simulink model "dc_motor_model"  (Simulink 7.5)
settings: Solver=ode45  StartTime=0.0  StopTime=40  RelTol=1e-3
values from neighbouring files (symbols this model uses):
  K = 12/4000    (= 0.003)    [INITIAL_PARAM.m]
  k2 = 12/4000    (= 0.003)    [INITIAL_PARAM.m]
  R = 10    [INITIAL_PARAM.m]
libraries: fl_lib x10, nesl_utility x4

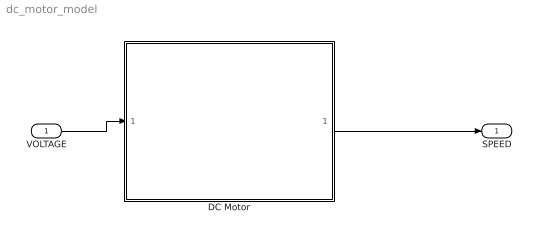
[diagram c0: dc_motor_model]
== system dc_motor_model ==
  VOLTAGE : Inport  OutDataType=fixdt(1, 16)  OutScaling=2^0
  DC Motor : Subsystem  mask{IMG='dcimaag.bmp'}
      mask prompts: IMG "Image File"
      mask init:
      | block=gcb;
      | img=imread(IMG);
  SPEED : Outport  OutDataType=fixdt(1, 16)  OutScaling=2^0
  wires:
  DC Motor/1(Speed) -> SPEED/1
  VOLTAGE/1 -> DC Motor/1(Voltage)

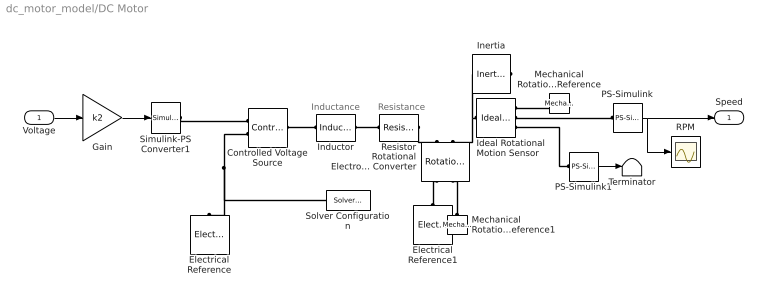
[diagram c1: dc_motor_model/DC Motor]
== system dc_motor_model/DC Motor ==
  note: Inductance
  note: Resistance
  Voltage : Inport  OutDataType=fixdt(1, 16)  OutScaling=2^0
  Controlled Voltage Source : fl_lib/Electrical/Electrical Sources/Controlled Voltage Source  DialogController=NetworkEngine.DynNeDlgSource  SystemSampleTime=-1  i_Log=off  v_Log=off  LocalVarNames=|i|v  LocalVarDescs=|i|v  LocalVarLogging=[0 0]
  Electrical Reference : fl_lib/Electrical/Electrical Elements/Electrical Reference  DialogController=NetworkEngine.DynNeDlgSource  SystemSampleTime=-1  i_Log=off  LocalVarNames=|i  LocalVarDescs=|i  LocalVarLogging=0
  Electrical Reference1 : fl_lib/Electrical/Electrical Elements/Electrical Reference  DialogController=NetworkEngine.DynNeDlgSource  SystemSampleTime=-1  i_Log=off  LocalVarNames=|i  LocalVarDescs=|i  LocalVarLogging=0
  Gain : Gain  Gain=k2  ParameterDataType=fixdt(1, 16)  ParameterScaling=2^0  OutDataType=fixdt(1, 16)  OutScaling=2^0
  Ideal Rotational Motion Sensor : fl_lib/Mechanical/Mechanical Sensors/Ideal Rotational Motion Sensor  DialogController=NetworkEngine.DynNeDlgSource  SystemSampleTime=-1  offset=0 deg  w_Log=off  t_Log=off  phi_Log=off  LocalVarNames=|w|t|phi  LocalVarDescs=|w|t|phi  LocalVarLogging=[]
  Inductor : fl_lib/Electrical/Electrical Elements/Inductor  DialogController=NetworkEngine.DynNeDlgSource  SystemSampleTime=-1  l=L mH  i0=0 A  r=0 Ohm  g=1e-9 1/Ohm  i_Log=off  v_Log=off  i_L_Log=off  LocalVarNames=|i|v|i_L  LocalVarDescs=|i|v|Internal variable for current through inductor term  LocalVarLogging=[0 0 0]
  Inertia : fl_lib/Mechanical/Rotational Elements/Inertia  DialogController=NetworkEngine.DynNeDlgSource  SystemSampleTime=-1  inertia=I kg*m^2  initial_velocity=0 rad/s  t_Log=off  LocalVarNames=|t  LocalVarDescs=|t  LocalVarLogging=0
  Mechanical Rotational Reference : fl_lib/Mechanical/Rotational Elements/Mechanical Rotational Reference  DialogController=NetworkEngine.DynNeDlgSource  SystemSampleTime=-1  t_Log=off  LocalVarNames=|t  LocalVarDescs=|t  LocalVarLogging=[]
  Mechanical Rotational Reference1 : fl_lib/Mechanical/Rotational Elements/Mechanical Rotational Reference  DialogController=NetworkEngine.DynNeDlgSource  SystemSampleTime=-1  t_Log=off  LocalVarNames=|t  LocalVarDescs=|t  LocalVarLogging=[]
  PS-Simulink : nesl_utility/PS-Simulink Converter  DialogController=NetworkEngine.DynNeUtilDlgSource  SystemSampleTime=-1  PhysicalDomain=network_engine_domain  LeftPortType=input  RightPortType=output  SubClassName=ps_output  Unit=rpm  AffineConversion=off
  PS-Simulink1 : nesl_utility/PS-Simulink Converter  DialogController=NetworkEngine.DynNeUtilDlgSource  SystemSampleTime=-1  PhysicalDomain=network_engine_domain  LeftPortType=input  RightPortType=output  SubClassName=ps_output  Unit=1  AffineConversion=off
  RPM : Scope
  Resistor : fl_lib/Electrical/Electrical Elements/Resistor  DialogController=NetworkEngine.DynNeDlgSource  SystemSampleTime=-1  R=R Ohm  i_Log=off  v_Log=off  LocalVarNames=|i|v  LocalVarDescs=|i|v  LocalVarLogging=[0 0]
  Rotational Electromechanical Converter : fl_lib/Electrical/Electrical Elements/Rotational Electromechanical Converter  DialogController=NetworkEngine.DynNeDlgSource  SystemSampleTime=-1  K=K V/rpm  i_Log=off  v_Log=off  t_Log=off  w_Log=off  LocalVarNames=|i|v|t|w  LocalVarDescs=|i|v|t|w  LocalVarLogging=[0 0 0 0]
  Simulink-PS Converter1 : nesl_utility/Simulink-PS Converter  DialogController=NetworkEngine.DynNeUtilDlgSource  SystemSampleTime=-1  PhysicalDomain=network_engine_domain  LeftPortType=input  RightPortType=output  SubClassName=ps_input  Unit=V  AffineConversion=off  InputFilterTimeConstant=.001  UdotUserProvided=0
  Solver Configuration : nesl_utility/Solver Configuration  DialogController=NetworkEngine.DynNeUtilDlgSource  SystemSampleTime=-1  PhysicalDomain=network_engine_domain  LeftPortType=input  RightPortType=generic  SubClassName=solver  Accelerate=off  Profile=off  ResidualTolerance=1e-9  MaxNonlinIter=3  MaxModeIter=2  DoFixedCost=off  UseLocalSampling=off  DoDC=off  LinearAlgebra=Sparse  LocalSolverSampleTime=.001  LocalSolverChoice=NE_BACKWARD_EULER_ADVANCER  UseLocalSolver=off
  Terminator : Terminator
  Speed : Outport  OutDataType=fixdt(1, 16)  OutScaling=2^0
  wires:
  PS-Simulink1/1 -> Terminator/1
  Voltage/1 -> Gain/1
  Gain/1 -> Simulink-PS Converter1/1
  PS-Simulink/1 -> Speed/1, RPM/1
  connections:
  Ideal Rotational Motion Sensor/LConn1 -- Rotational Electromechanical Converter/LConn2 -- Inertia/LConn1
  Inductor/RConn1 -- Resistor/LConn1
  Resistor/RConn1 -- Rotational Electromechanical Converter/LConn1
  PS-Simulink1/LConn1 -- Ideal Rotational Motion Sensor/RConn3
  Controlled Voltage Source/LConn1 -- Inductor/LConn1
  Simulink-PS Converter1/RConn1 -- Controlled Voltage Source/RConn1
  Electrical Reference1/LConn1 -- Rotational Electromechanical Converter/RConn1
  PS-Simulink/LConn1 -- Ideal Rotational Motion Sensor/RConn2
  Controlled Voltage Source/RConn2 -- Electrical Reference/LConn1 -- Solver Configuration/RConn1
  Mechanical Rotational Reference/LConn1 -- Ideal Rotational Motion Sensor/RConn1
  Mechanical Rotational Reference1/LConn1 -- Rotational Electromechanical Converter/RConn2
